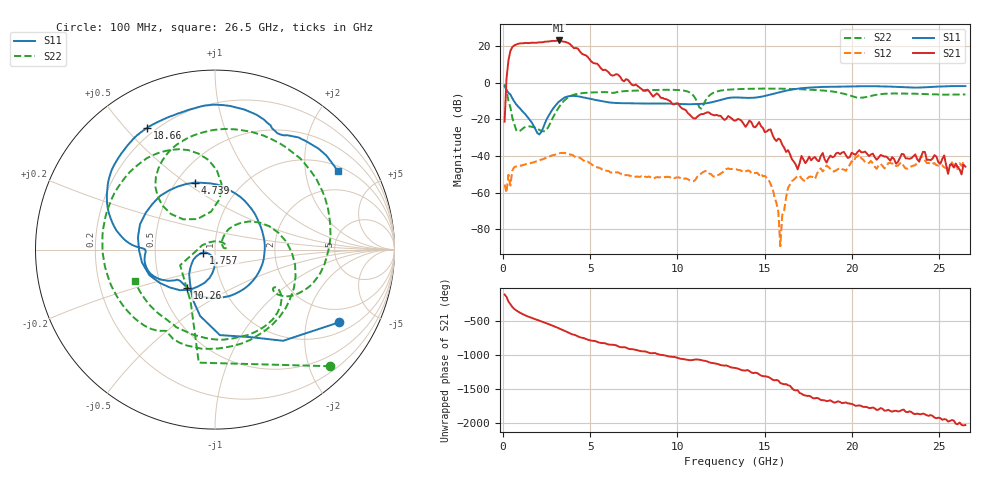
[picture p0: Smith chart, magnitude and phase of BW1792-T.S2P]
!Agilent Technologies,N5242A,MY48420835,A.09.90.17
!Agilent N5242A: A.09.90.17
!Date: Monday, August 22, 2016 14:00:26
!Correction: S11(Full 2 Port(1,2))
!S21(Full 2 Port(1,2))
!S12(Full 2 Port(1,2))
!S22(Full 2 Port(1,2))
!S2P File: Measurements: S11, S21, S12, S22:
# Hz S  dB  R 50
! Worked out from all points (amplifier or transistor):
!   240 points, 100 MHz to 26.5 GHz, reference 50 ohm
!   highest |S21| = 23.1 dB at 3.193 GHz (marker M1)
!   |S21| within 3 dB of that: 614.1 MHz to 3.949 GHz (3.334 GHz wide, 146 % of centre)
!   unconditionally stable (mu >= 1): start of sweep to end of sweep
!   at 4.518 GHz: K = 6.02, MAG = 18.0 dB, |S12| = -41.7 dB
!   at 13.36 GHz: K = 570.25, MAG = -17.2 dB, |S12| = -47.2 dB
!   at 26.5 GHz: K = 4127.85, MAG = -40.0 dB, |S12| = -44.1 dB
!   S11 on the Smith chart (normalised r, x): 100 MHz: 1.38, -3.11; 1.757 GHz: 0.88, -0.03; 4.739 GHz: 0.62, +0.54; 10.26 GHz: 0.68, -0.31; 18.66 GHz: 0.17, +0.57; 26.5 GHz: 1.17, +3.00
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1e8  -1.94 -30.4  -21.20 -104.8  -55.60 22.7  -0.78 -45.3
3.209205e8  -5.56 -67.8  12.29 151.0  -50.25 18.5  -9.90 -115.1
5.41841e8  -8.42 -102.6  19.50 72.6  -47.93 61.1  -19.11 -173.8
7.627615e8  -11.75 -121.4  20.87 22.0  -45.72 31.2  -25.83 127.1
9.83682e8  -14.04 -136.5  21.49 -13.6  -45.26 19.3  -26.26 70.2
1.315063e9  -17.50 -154.8  21.77 -54.9  -44.46 8.5  -24.00 29.1
1.756904e9  -23.37 -166.2  21.84 -100.3  -43.44 -1.9  -24.22 8.4
2.530126e9  -19.54 -92.6  22.50 -172.2  -40.79 -25.4  -25.23 43.8
2.861506e9  -14.30 -107.1  22.85 155.3  -39.50 -39.6  -19.13 57.8
3.192887e9  -10.50 -130.6  23.09 119.9  -38.56 -58.3  -13.62 45.8
3.524268e9  -8.11 -158.9  22.38 82.1  -38.26 -80.6  -9.63 23.2
3.855649e9  -7.23 171.0  21.03 41.6  -39.17 -100.9  -7.35 -2.5
4.51841e9  -7.78 120.8  15.96 -20.9  -41.68 -138.9  -5.69 -46.1
4.739331e9  -8.18 106.7  15.08 -36.7  -43.08 -144.9  -5.50 -58.1
6.064854e9  -10.69 36.4  5.63 -121.6  -48.24 176.6  -5.19 -115.0
8.93682e9  -11.34 -90.5  -6.67 93.0  -51.63 80.0  -3.89 160.3
1.026234e10  -11.64 -126.1  -14.00 27.2  -52.66 28.9  -4.13 118.9
1.335523e10  -8.01 -170.0  -20.53 -109.4  -47.22 -87.1  -3.51 90.2
1.777364e10  -2.53 134.3  -41.16 166.5  -51.59 169.9  -3.86 3.7
1.865732e10  -2.20 119.3  -41.38 130.5  -46.01 114.5  -4.49 -13.9
2.219205e10  -2.10 72.6  -42.57 -19.1  -43.75 -27.9  -5.88 -55.3
2.65e10  -1.82 32.6  -45.79 132.9  -44.14 84.3  -6.39 -158.9
